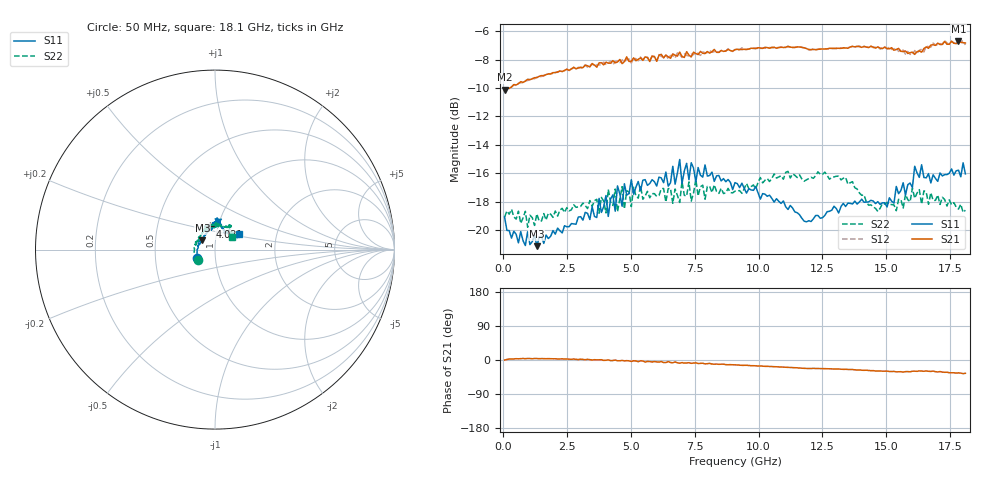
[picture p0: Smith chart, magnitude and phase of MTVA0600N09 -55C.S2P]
! Network Analyzer HP8720D.06.14 Serial No. US36140669
!  7 Jul 2005  06:35:05
! Frequency  S11  S21  S12  S22
# HZ  S  DB R 50
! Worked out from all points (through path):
!   201 points, 50 MHz to 18.1 GHz, reference 50 ohm
!   highest |S21| = -6.71 dB at 17.83 GHz (marker M1); lowest = -10.1 dB at 50 MHz (marker M2)
!   group delay of S21, straight-line fit = 6.61 ps
!   lowest |S11| = -21.1 dB at 1.313 GHz (marker M3), VSWR 1.19, Z = 43.2 + j4.59 ohm
!   |S11| at or under -10 dB: start of sweep to end of sweep
!   |S22| runs from -19.8 to -15.9 dB; largest |S21 - S12| = 0.017
!   S11 on the Smith chart (normalised r, x): 50 MHz: 0.81, -0.08; 4.021 GHz: 0.91, +0.24; 18.1 GHz: 1.28, +0.23
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5e7  -19.08 -154.3  -10.13 -0.1  -10.15 0.1  -19.07 -148.6
1.3135e9  -21.11 143.1  -9.27 3.9  -9.23 3.6  -18.85 143.6
3.1185e9  -19.29 111.5  -8.57 1.6  -8.60 1.2  -18.08 122.8
4.021e9  -17.56 102.7  -8.19 -0.7  -8.34 0.4  -18.78 114.0
4.11125e9  -19.02 101.0  -8.25 0.4  -8.23 -1.2  -17.12 112.5
4.47225e9  -16.88 92.4  -8.17 -2.0  -8.12 -0.4  -18.69 115.9
4.65275e9  -18.31 91.7  -8.29 -1.1  -8.02 -1.9  -16.93 114.1
4.743e9  -16.73 94.5  -8.15 -2.4  -8.18 -1.2  -18.50 109.8
5.104e9  -17.46 95.5  -7.88 -2.0  -7.91 -3.2  -16.97 104.4
6.09675e9  -16.26 87.7  -7.70 -5.4  -7.65 -5.2  -17.55 98.5
6.7285e9  -16.75 89.6  -7.69 -5.1  -7.91 -6.1  -17.10 90.4
6.909e9  -15.03 86.4  -7.48 -8.5  -7.65 -7.0  -18.04 87.3
6.99925e9  -16.72 85.8  -7.78 -6.9  -7.86 -8.5  -16.58 88.3
7.36025e9  -15.25 78.2  -7.82 -8.8  -7.62 -7.6  -17.95 90.7
7.54075e9  -16.60 78.9  -7.58 -7.4  -7.45 -9.6  -16.42 88.5
9.075e9  -16.65 80.1  -7.31 -12.8  -7.29 -12.9  -17.25 69.3
1.21435e10  -19.20 60.3  -7.29 -22.1  -7.25 -22.2  -16.35 60.0
1.512175e10  -17.72 27.6  -7.25 -30.4  -7.10 -30.2  -18.20 48.8
1.602425e10  -17.00 31.0  -7.49 -29.6  -7.67 -31.1  -17.04 45.0
1.61145e10  -15.50 30.0  -7.64 -29.4  -7.37 -29.7  -17.75 46.4
1.782925e10  -15.77 36.3  -6.71 -33.9  -6.78 -33.2  -18.51 39.8
1.81e10  -16.04 33.9  -6.84 -35.1  -6.97 -35.4  -18.59 37.7
